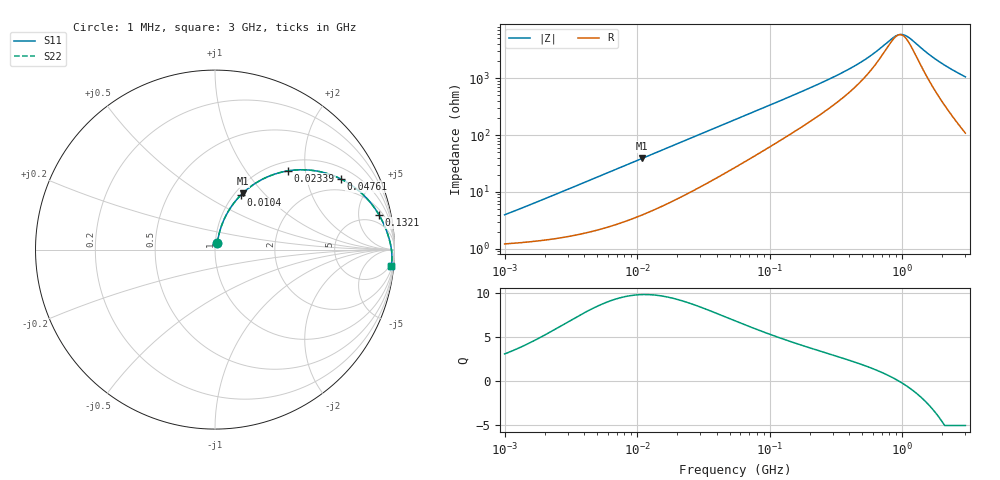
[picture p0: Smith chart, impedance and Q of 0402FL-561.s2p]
# MHz S MA R 50
!Freq  MagS11  AngS11  MagS21  AngS21  MagS12  AngS12  MagS22  AngS22
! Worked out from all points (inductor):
!   801 points, 1 MHz to 3 GHz, reference 50 ohm
!   read as one part in series: L = 595 nH near 1.041 MHz
!   highest Q = 9.82 at 10.93 MHz (marker M1), where L = 562 nH
!   self-resonance near 949.9 MHz
!   S11 on the Smith chart (normalised r, x): 1 MHz: 1.02, +0.08; 10.4 MHz: 1.08, +0.74; 23.39 MHz: 1.18, +1.62; 47.61 MHz: 1.44, +3.21; 132.1 MHz: 2.83, +8.60; 3 GHz: 3, -21
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1  0.03903 70.0  0.9873 -2.1  0.9873 -2.1  0.03903 70.0
2.076287  0.07671 75.1  0.9831 -4.3  0.9831 -4.3  0.07671 75.1
3.823119  0.1365 74.7  0.973 -7.8  0.973 -7.8  0.1365 74.7
6.629334  0.227 70.8  0.9498 -13.0  0.9498 -13.0  0.227 70.8
10.40059  0.3361 64.6  0.9083 -19.5  0.9083 -19.5  0.3361 64.6
10.93427  0.3503 63.8  0.9018 -20.4  0.9018 -20.4  0.3503 63.8
14.47069  0.4365 58.4  0.8561 -25.7  0.8561 -25.7  0.4365 58.4
23.39465  0.5991 47.1  0.7371 -36.5  0.7371 -36.5  0.5991 47.1
32.87715  0.7078 38.4  0.6258 -44.6  0.6258 -44.6  0.7078 38.4
47.61141  0.8031 29.4  0.4957 -52.7  0.4957 -52.7  0.8031 29.4
54.77226  0.8317 26.3  0.448 -55.4  0.448 -55.4  0.8317 26.3
82.55875  0.8932 18.5  0.3227 -61.7  0.3227 -61.7  0.8932 18.5
132.1429  0.9338 12.0  0.2125 -66.0  0.2125 -66.0  0.9338 12.0
209.4008  0.9557 7.6  0.1365 -67.3  0.1365 -67.3  0.9557 7.6
328.5236  0.9682 4.6  0.08455 -65.7  0.08455 -65.7  0.9682 4.6
461.6833  0.9746 2.9  0.05536 -61.2  0.05536 -61.2  0.9746 2.9
604.9187  0.9784 1.7  0.0366 -53.0  0.0366 -53.0  0.9784 1.7
792.5923  0.9814 0.7  0.02192 -31.7  0.02192 -31.7  0.9814 0.7
930.2341  0.9829 0.1  0.01716 -4.5  0.01716 -4.5  0.9829 0.1
1059.487  0.9839 -0.4  0.01754 23.5  0.01754 23.5  0.9839 -0.4
1837.163  0.9867 -2.7  0.04797 72.6  0.04797 72.6  0.9867 -2.7
3000  0.986 -5.4  0.09377 78.8  0.09377 78.8  0.986 -5.4
